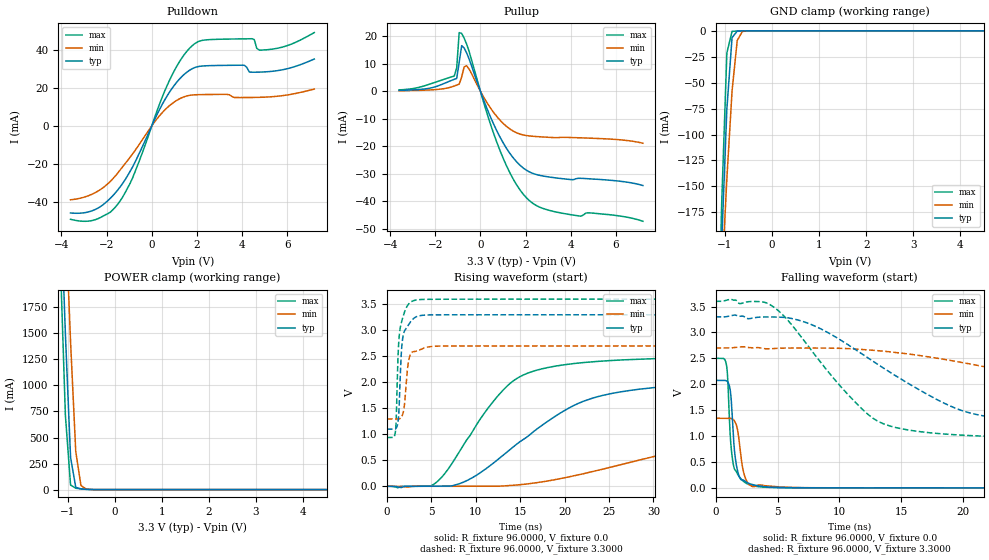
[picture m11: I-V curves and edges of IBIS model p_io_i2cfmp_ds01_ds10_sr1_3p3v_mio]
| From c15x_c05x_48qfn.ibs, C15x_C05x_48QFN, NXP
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[Model] p_io_i2cfmp_ds01_ds10_sr1_3p3v_mio
|   Model p_io_i2cfmp_ds01_ds10_sr1_3p3v_mio
| This model was characterised for following simulation conditions:
| External (pad) voltage:
|   - Typ: 3.3V,   - Min: 2.7V,   - Max: 3.6V
| Library cells for typ/min/max conditions are connected as defined below:
|  pad - External Pad
|  ipp_do_lv - Core Input
|  ipp_obe_lv - Output Buffer Enable
|  IOGC - NC
|  REFH3V3 - REFH3V3
|  REFL3V3 - REFL3V3
|  ZI - NC
|  abut_ncal_vddio[1] - vddio
|  abut_ncal_vddio[2] - vddio
|  abut_ncal_vddio[3] - vssio
|  abut_ncal_vddio[4] - vddio
|  abut_ncal_vddio[5] - vddio
|  abut_ncal_vddio[6] - vssio
|  abut_pcal_vddio[1] - vssio
|  abut_pcal_vddio[2] - vssio
|  abut_pcal_vddio[3] - vddio
|  abut_pcal_vddio[4] - vssio
|  abut_pcal_vddio[5] - vssio
|  abut_pcal_vddio[6] - vddio
|  ipp_do_1p8v - ipp_do_1p8v
|  ipp_dse_lv[0] - vdd_lv
|  ipp_dse_lv[1] - 0
|  ipp_eftd_lv - NC
|  ipp_ina_mux_vddio - NC
|  ipp_ina_mux_vddio[0] - NC
|  ipp_ina_mux_vddio[1] - NC
|  ipp_ina_r0_vddio - NC
|  ipp_ina_r0a_vddio - NC
|  ipp_ina_r0b_vddio - NC
|  ipp_ina_r0c_vddio - NC
|  ipp_ina_r0d_vddio - NC
|  ipp_ina_r0e_vddio - NC
|  ipp_ina_r0f_vddio - NC
|  ipp_ina_r300_vddio - NC
|  ipp_ina_r300a_vddio - NC
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Model_type I/O
Polarity   Non-Inverting
Enable   Active-High
Vinl =   0.9900V
Vinh =   2.3100V
Vmeas =  1.6500V
Cref =   30.0000pF
Rref =   1.0000M
Vref =   3.3000V
C_comp   1.7403pF   1.7015pF   1.7922pF
|C_comp_pullup   0.6950pF   0.7586pF   0.6579pF
|C_comp_pulldown   0.9320pF   0.9171pF   0.9310pF
[Model Spec]
| variable   typ   min   max
Vinh   2.3100V   1.8900V   2.5200V
Vinl   0.9900V   0.8100V   1.0800V
[Temperature Range]   25.0000   0.1250k   -40.0000
[Voltage Range]   3.3000V   2.7000V   3.6000V
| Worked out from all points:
|   slope of the pulldown table from 0 to 0.495 V, typ, clamps not added: 41.2 ohm
|   slope of the pullup table from 0 to 0.495 V, typ, clamps not added: 48.1 ohm
|   GND clamp passes 1 mA (typ) near -0.75 V on its own axis
|   POWER clamp passes 1 mA (typ) near -0.52 V on its own axis
|   rising waveform, R_fixture 96.0000, V_fixture 0.0: 20-80 % time 10.8ns typ, 22.9ns min, 6.46ns max; typ from 0 V to 2.08 V
|   rising waveform, R_fixture 96.0000, V_fixture 3.3000: 20-80 % time 409ps typ, 472ps min, 441ps max; typ from 1.1 V to 3.3 V
|   falling waveform, R_fixture 96.0000, V_fixture 0.0: 20-80 % time 423ps typ, 491ps min, 395ps max; typ from 2.08 V to 0 V
|   falling waveform, R_fixture 96.0000, V_fixture 3.3000: 20-80 % time 9.3ns typ, 20.2ns min, 5.64ns max; typ from 3.3 V to 1.1 V
[Pulldown]
|Voltage   I(typ)   I(min)   I(max)
-3.6V     -45.91mA   -38.97mA   -49.24mA
-2.5V     -44.06mA   -35.15mA   -49.44mA
-1.4V     -32.16mA   -23.22mA   -39.53mA
-850mV    -21.66mA   -14.77mA   -27.43mA
800mV     18.06mA    10.83mA    24.4mA
1.35V     26.21mA    14.95mA    36.11mA
1.9V      30.74mA    16.39mA    43.35mA
4.1V      31.97mA    14.95mA    45.9mA
4.43V     28.32mA    14.99mA    45.97mA
4.65V     28.33mA    15.03mA    40.92mA
5.09V     28.54mA    15.22mA    40.14mA
7.2V      35.25mA    19.41mA    49.21mA
[Pullup]
|Voltage   I(typ)   I(min)   I(max)
-3.6V     311.2uA    185.3uA    486.9uA
-1.16V    4.313mA    1.883mA    5.48mA
-1.05V    4.647mA    2.223mA    8.477mA
-940mV    10.46mA    2.573mA    21.3mA
-830mV    16.55mA    5.158mA    20.99mA
-720mV    15.7mA     8.801mA    19.26mA
-610mV    13.89mA    9.254mA    17.11mA
820mV     -15.89mA   -10.08mA   -20.54mA
1.48V     -24.47mA   -14.6mA    -32.29mA
2.03V     -28.65mA   -16.09mA   -38.62mA
3.46V     -31.6mA    -16.83mA   -44.04mA
7.2V      -34.25mA   -18.88mA   -47.24mA
[GND_clamp]
|Voltage   I(typ)   I(min)   I(max)
-3.6V     -4.377A    -3.283A    -5.855A
-1.18V    -351.7mA   -346.5mA   -367.9mA
-1.07V    -204.2mA   -241.2mA   -166.2mA
-960mV    -75.42mA   -142.6mA   -21.4mA
-850mV    -6.575mA   -58.21mA   -529.8uA
-740mV    -281.6uA   -9.383mA   -183.8uA
-630mV    -73.66uA   -605.1uA   -74.76uA
-410mV    -3.148uA   -9.219uA   -1.868uA
7.2V      0A         0A         0A
[POWER_clamp]
|Voltage   I(typ)   I(min)   I(max)
-3.6V     34.56A     31.8A      37.41A
-1.16V    2.902A     3.904A     2.233A
-1.05V    1.495A     2.658A     715.5mA
-940mV    310.6mA    1.419A     44.07mA
-830mV    22.38mA    368.3mA    13.28mA
-720mV    6.713mA    39.84mA    7.005mA
-610mV    2.702mA    5.591mA    2.612mA
7.2V      0A         0A         0A
[Ramp]
| variable   typ   min   max
dV/dt_r  1.2449/10.7748n   0.8034/22.9369n   1.5004/6.4590n
dV/dt_f  1.3207/9.2987n   0.8413/20.2416n   1.5974/5.6388n
R_load = 96.0000
[Rising Waveform]
R_fixture= 96.0000
V_fixture= 0.0
V_fixture_min= 0.0
V_fixture_max= 0.0
|time   V(typ)   V(min)   V(max)
0s        3.929nV    315.7nV    13.68nV
5.055ns   -157.3uV   -370.6uV   16.44mV
8.639ns   80.53mV    -57.75uV   804.3mV
11.65ns   401.3mV    613.1uV    1.563V
14.2ns    754.9mV    18.26mV    2.025V
21.06ns   1.556V     201.2mV    2.361V
30.64ns   1.907V     597.8mV    2.457V
41.09ns   2.006V     973.7mV    2.486V
52.44ns   2.046V     1.159V     2.496V
134.5ns   2.075V     1.339V     2.501V
[Rising Waveform]
R_fixture= 96.0000
V_fixture= 3.3000
V_fixture_min= 2.7000
V_fixture_max= 3.6000
|time   V(typ)   V(min)   V(max)
0s        1.099V     1.294V     937.7mV
958.9ps   1.104V     1.294V     1.056V
1.045ns   1.119V     1.294V     1.299V
1.21ns    1.203V     1.294V     2.324V
1.307ns   1.335V     1.294V     2.715V
1.563ns   2.39V      1.315V     3.105V
1.852ns   2.924V     1.435V     3.286V
2.509ns   3.127V     2.468V     3.519V
3.485ns   3.272V     2.609V     3.588V
134.5ns   3.3V       2.7V       3.6V
[Falling Waveform]
R_fixture= 96.0000
V_fixture= 0.0
V_fixture_min= 0.0
V_fixture_max= 0.0
|time   V(typ)   V(min)   V(max)
0s        2.075V     1.344V     2.501V
873.5ps   2.068V     1.343V     2.381V
977.2ps   2.046V     1.343V     2.117V
1.206ns   1.846V     1.342V     925.4mV
1.517ns   742.5mV    1.294V     370.2mV
1.897ns   227.6mV    919.7mV    219.9mV
2.179ns   152.2mV    392.8mV    142.3mV
2.457ns   113.9mV    159.2mV    90.57mV
3.776ns   28.13mV    49.57mV    15.37mV
134.5ns   167.1nV    3.515uV    25.61nV
[Falling Waveform]
R_fixture= 96.0000
V_fixture= 3.3000
V_fixture_min= 2.7000
V_fixture_max= 3.6000
|time   V(typ)   V(min)   V(max)
0s        3.3V       2.7V       3.6V
4.395ns   3.299V     2.684V     3.536V
8.034ns   3.122V     2.699V     2.562V
12.65ns   2.454V     2.657V     1.354V
18.03ns   1.685V     2.498V     1.047V
21.01ns   1.419V     2.371V     1.004V
26.25ns   1.259V     2.123V     968.5mV
37.37ns   1.154V     1.647V     945.8mV
48.07ns   1.123V     1.466V     940.4mV
134.5ns   1.099V     1.298V     937.7mV
